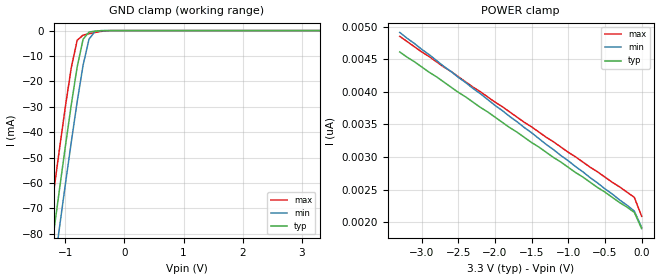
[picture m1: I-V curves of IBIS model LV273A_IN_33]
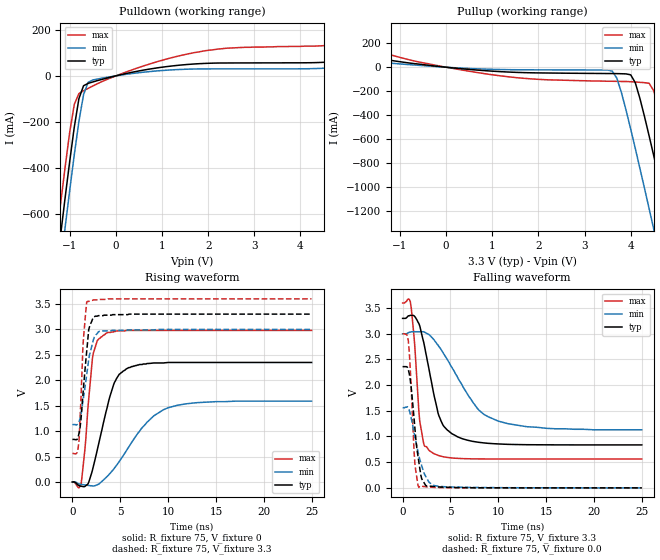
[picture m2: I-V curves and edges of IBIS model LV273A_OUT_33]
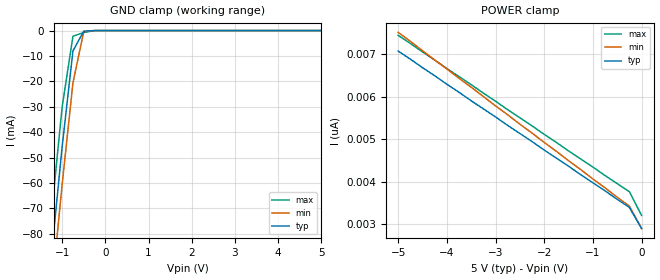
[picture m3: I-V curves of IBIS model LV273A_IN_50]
| TEXAS INSTRUMENTS INCORPORATED
| Standard Linear and Logic Group
| IBIS Model of SN74LV273A
| OCTAL EDGE-TRIGGERED D-TYPE FLIP-FLOP WITH CLEAR
| SOIC 20-pin (DW), SOP 20-pin (NS), SSOP 20-pin (DB), TSSOP 20-pin (PW)
| and TVSOP 20-pin (DGV) Package
[IBIS Ver]   3.2
[Comment Char]  |_char
[File Name]   lv273a.ibs
[File Rev]   2.0 H_die
[Date]   May 29, 2000
[Source]   Data created from HSPICE simulations at TI-SLL.
[Notes]   The following is an IBIS list for the LV273A.
|   Please contact sllibis@ti.com with questions and
|   comments concerning SLL IBIS models.
[Disclaimer] Property of Texas Instruments Incorporated.  Unauthorized
   reproduction and/or distribution is strictly prohibited.
   This product is protected under copyright law.
   Created 2000, (C) Copyright 2000, Texas Instruments Inc.,
   All Rights Reserved.
   UNLESS THERE IS A SIGNED, WRITTEN AGREEMENT TO THE
   CONTRARY, TEXAS INSTRUMENTS () IS PROVIDING THE IBIS
   MODELS  AND WITHOUT ANY WARRANTY, EXPRESSED OR
   IMPLIED.  TI assumes no liability for:
   1) the accuracy of the IBIS models provided to your
   company;
   2) the proper functioning of these IBIS Models in your
   design or for any resulting applications; or
   3) infringement of patents, copyrights or intellectual
   property rights resulting from your use of these IBIS
   models.
   TI provides IBIS Models as a service to our customers.
   You and your company shall not distribute, sell or give
   these models to anyone else without prior written
   permission from TI.
   TI reserves the right to make changes to our products or
   to discontinue any semiconductor product or service
   without notice, and advises our customers to obtain the
   latest version of relevant information to verify, before
   placing orders, that the information being relied on is
   current.
   Please be aware that your receipt and use of the IBIS
   information provided shall serve as acceptance of these
   terms and conditions.  If you do not accept these terms,
   you should return or destroy the IBIS models and any
   other accompanying information immediately.
|   Component LV273A_DW
[Component]   LV273A_DW
[Manufacturer]  Texas Instruments, Inc.
[Package]
|   typ   min   max
R_pkg   0.038   0.033   0.045
L_pkg   5.012nH   4.110nH   6.349nH
C_pkg   0.717pF   0.530pF   0.868pF
[Pin]   signal_name   model_name   R_pin   L_pin   C_pin
1   CLR_NOT   LV273A_IN   0.042   6.336nH   0.865pF
2   1Q   LV273A_OUT   0.043   5.542nH   0.867pF
3   1D   LV273A_IN   0.034   4.714nH   0.732pF
4   2D   LV273A_IN   0.034   4.377nH   0.591pF
5   2Q   LV273A_OUT   0.036   4.130nH   0.533pF
6   3Q   LV273A_OUT   0.035   4.111nH   0.530pF
7   3D   LV273A_IN   0.034   4.284nH   0.583pF
8   4D   LV273A_IN   0.034   4.634nH   0.726pF
9   4Q   LV273A_OUT   0.040   5.518nH   0.865pF
10   GND   GND   0.043   6.349nH   0.866pF
11   CLK   LV273A_IN   0.041   6.281nH   0.861pF
12   5Q   LV273A_OUT   0.045   5.561nH   0.868pF
13   5D   LV273A_IN   0.033   4.778nH   0.742pF
14   6D   LV273A_IN   0.035   4.414nH   0.596pF
15   6Q   LV273A_OUT   0.035   4.110nH   0.533pF
16   7Q   LV273A_OUT   0.036   4.130nH   0.533pF
17   7D   LV273A_IN   0.034   4.377nH   0.591pF
18   8D   LV273A_IN   0.034   4.714nH   0.731pF
19   8Q   LV273A_OUT   0.043   5.569nH   0.868pF
20   VCC   POWER   0.042   6.308nH   0.864pF
|   Component LV273A_NS
[Component]   LV273A_NS
[Manufacturer]  Texas Instruments, Inc.
[Package]
|   typ   min   max
R_pkg   0.044   0.029   0.058
L_pkg   3.666nH   2.317nH   5.115nH
C_pkg   0.548pF   0.316pF   0.725pF
[Pin]   signal_name   model_name   R_pin   L_pin   C_pin
1   CLR_NOT   LV273A_IN   0.058   5.115nH   0.725pF
2   1Q   LV273A_OUT   0.053   4.591nH   0.724pF
3   1D   LV273A_IN   0.049   3.754nH   0.572pF
4   2D   LV273A_IN   0.029   2.549nH   0.388pF
5   2Q   LV273A_OUT   0.031   2.317nH   0.316pF
6   3Q   LV273A_OUT   0.031   2.317nH   0.316pF
7   3D   LV273A_IN   0.029   2.556nH   0.399pF
8   4D   LV273A_IN   0.049   3.754nH   0.579pF
9   4Q   LV273A_OUT   0.053   4.591nH   0.724pF
10   GND   GND   0.058   5.115nH   0.725pF
11   CLK   LV273A_IN   0.058   5.115nH   0.725pF
12   5Q   LV273A_OUT   0.053   4.591nH   0.724pF
13   5D   LV273A_IN   0.049   3.754nH   0.579pF
14   6D   LV273A_IN   0.029   2.557nH   0.399pF
15   6Q   LV273A_OUT   0.031   2.317nH   0.316pF
16   7Q   LV273A_OUT   0.031   2.317nH   0.316pF
17   7D   LV273A_IN   0.029   2.557nH   0.399pF
18   8D   LV273A_IN   0.049   3.754nH   0.579pF
19   8Q   LV273A_OUT   0.053   4.591nH   0.724pF
20   VCC   POWER   0.058   5.115nH   0.725pF
|   Component LV273A_DB
[Component]   LV273A_DB
[Manufacturer]  Texas Instruments, Inc.
[Package]
|   typ   min   max
R_pkg   0.040   0.035   0.051
L_pkg   3.495nH   3.035nH   4.314nH
C_pkg   0.420pF   0.346pF   0.502pF
[Pin]   signal_name   model_name   R_pin   L_pin   C_pin
1   CLR_NOT   LV273A_IN   0.049   4.310nH   0.502pF
2   1Q   LV273A_OUT   0.048   3.903nH   0.487pF
3   1D   LV273A_IN   0.035   3.189nH   0.396pF
4   2D   LV273A_IN   0.035   3.036nH   0.347pF
5   2Q   LV273A_OUT   0.035   3.035nH   0.367pF
6   3Q   LV273A_OUT   0.035   3.035nH   0.367pF
7   3D   LV273A_IN   0.035   3.036nH   0.347pF
8   4D   LV273A_IN   0.035   3.189nH   0.397pF
9   4Q   LV273A_OUT   0.047   3.899nH   0.488pF
10   GND   GND   0.051   4.314nH   0.500pF
11   CLK   LV273A_IN   0.051   4.314nH   0.500pF
12   5Q   LV273A_OUT   0.047   3.899nH   0.488pF
13   5D   LV273A_IN   0.035   3.189nH   0.397pF
14   6D   LV273A_IN   0.035   3.036nH   0.346pF
15   6Q   LV273A_OUT   0.035   3.035nH   0.367pF
16   7Q   LV273A_OUT   0.035   3.035nH   0.367pF
17   7D   LV273A_IN   0.035   3.036nH   0.346pF
18   8D   LV273A_IN   0.035   3.189nH   0.397pF
19   8Q   LV273A_OUT   0.047   3.899nH   0.488pF
20   VCC   POWER   0.051   4.314nH   0.502pF
|   Component LV273A_PW
[Component]   LV273A_PW
[Manufacturer]  Texas Instruments, Inc.
[Package]
|   typ   min   max
R_pkg   0.035   0.024   0.047
L_pkg   2.399nH   1.710nH   3.250nH
C_pkg   0.284pF   0.166pF   0.418pF
[Pin]   signal_name   model_name   R_pin   L_pin   C_pin
1   CLR_NOT   LV273A_IN   0.041   3.102nH   0.410pF
2   1Q   LV273A_OUT   0.040   2.777nH   0.363pF
3   1D   LV273A_IN   0.029   2.194nH   0.260pF
4   2D   LV273A_IN   0.025   1.710nH   0.166pF
5   2Q   LV273A_OUT   0.025   1.740nH   0.191pF
6   3Q   LV273A_OUT   0.024   1.763nH   0.193pF
7   3D   LV273A_IN   0.024   1.817nH   0.174pF
8   4D   LV273A_IN   0.028   2.256nH   0.265pF
9   4Q   LV273A_OUT   0.045   2.887nH   0.368pF
10   GND   GND   0.047   3.250nH   0.417pF
11   CLK   LV273A_IN   0.046   3.244nH   0.418pF
12   5Q   LV273A_OUT   0.046   2.961nH   0.375pF
13   5D   LV273A_IN   0.033   2.334nH   0.268pF
14   6D   LV273A_IN   0.029   1.915nH   0.179pF
15   6Q   LV273A_OUT   0.031   1.934nH   0.203pF
16   7Q   LV273A_OUT   0.032   1.917nH   0.201pF
17   7D   LV273A_IN   0.030   1.833nH   0.173pF
18   8D   LV273A_IN   0.036   2.324nH   0.268pF
19   8Q   LV273A_OUT   0.042   2.869nH   0.372pF
20   VCC   POWER   0.042   3.160nH   0.414pF
|   Component LV273A_DGV
[Component]   LV273A_DGV
[Manufacturer]  Texas Instruments, Inc.
[Package]
|   typ   min   max
R_pkg   0.044   0.038   0.048
L_pkg   2.561nH   2.236nH   2.961nH
C_pkg   0.342pF   0.264pF   0.446pF
[Pin]   signal_name   model_name   R_pin   L_pin   C_pin
1   CLR_NOT   LV273A_IN   0.044   2.935nH   0.417pF
2   1Q   LV273A_OUT   0.042   2.869nH   0.446pF
3   1D   LV273A_IN   0.043   2.399nH   0.316pF
4   2D   LV273A_IN   0.044   2.236nH   0.265pF
5   2Q   LV273A_OUT   0.046   2.278nH   0.264pF
6   3Q   LV273A_OUT   0.045   2.274nH   0.264pF
7   3D   LV273A_IN   0.044   2.285nH   0.269pF
8   4D   LV273A_IN   0.043   2.452nH   0.320pF
9   4Q   LV273A_OUT   0.044   2.900nH   0.446pF
10   GND   GND   0.044   2.961nH   0.418pF
11   CLK   LV273A_IN   0.045   2.954nH   0.418pF
12   5Q   LV273A_OUT   0.042   2.847nH   0.443pF
13   5D   LV273A_IN   0.045   2.453nH   0.319pF
14   6D   LV273A_IN   0.045   2.297nH   0.269pF
15   6Q   LV273A_OUT   0.048   2.334nH   0.268pF
16   7Q   LV273A_OUT   0.048   2.335nH   0.267pF
17   7D   LV273A_IN   0.046   2.299nH   0.268pF
18   8D   LV273A_IN   0.046   2.457nH   0.320pF
19   8Q   LV273A_OUT   0.043   2.848nH   0.441pF
20   VCC   POWER   0.038   2.812nH   0.408pF
[Model Selector]   LV273A_IN
LV273A_IN_33   3.3-V Vcc Input Model
LV273A_IN_50   5.0-V Vcc Input Model
[Model Selector]   LV273A_OUT
LV273A_OUT_33   3.3-V Vcc Output Model
LV273A_OUT_50   5.0-V Vcc Output Model
| Models and submodels in the file (4): LV273A_IN_33 (Input), LV273A_OUT_33 (Output), LV273A_IN_50 (Input), LV273A_OUT_50 (Output)
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|   Model LV273A_IN_33
[Model]   LV273A_IN_33
Model_type  Input
Polarity   Inverting
Vinl = 0.99
Vinh = 2.31
| variable   typ   min   max
C_comp   1.43pf   1.07pf   1.79pf
[Temperature Range]   25   85   -40
[Voltage Range]   3.3   3.0   3.6
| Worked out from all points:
|   GND clamp passes 1 mA (typ) near -0.61 V on its own axis
[GND Clamp]
|   Voltage   I(typ)   I(min)   I(max)
-3.3V     -460mA     -475mA     -445mA
-1.3V     -97.5mA    -113mA     -81.5mA
-1.2V     -79.9mA    -95mA      -63.9mA
-1.1V     -62.6mA    -77.6mA    -46.7mA
-1V       -45.6mA    -60.5mA    -30mA
-900mV    -29.2mA    -43.9mA    -14.6mA
-800mV    -14.3mA    -28mA      -3.81mA
-700mV    -3.42mA    -13.6mA    -1.78mA
-600mV    -581uA     -3.4mA     -1.25mA
-500mV    -233uA     -353uA     -759uA
-400mV    -58.1uA    -21.9uA    -324uA
3.3V      1.9nA      2.34nA     1.69nA
[POWER Clamp]
|   Voltage   I(typ)   I(min)   I(max)
-3.3V     4.61nA     4.91nA     4.85nA
-3V       4.38nA     4.65nA     4.61nA
-100mV    2.15nA     2.17nA     2.38nA
0V        1.9nA      1.92nA     2.09nA
|   Model LV273A_OUT_33
[Model]   LV273A_OUT_33
Model_type  Output
Polarity   Non-Inverting
Vmeas = 1.65v
Cref = 15pf
| variable   typ   min   max
C_comp   7.60pf   5.70pf   9.50pf
[Temperature Range]   25   85   -40
[Voltage Range]   3.3   3.0   3.6
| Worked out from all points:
|   slope of the pulldown table from 0 to 0.495 V, typ, clamps not added: 23.3 ohm
|   slope of the pullup table from 0 to 0.495 V, typ, clamps not added: 27.2 ohm
|   rising waveform, R_fixture 75, V_fixture 0: 20-80 % time 1.85ns typ, 3.78ns min, 791ps max; typ from 0 V to 2.35 V
|   falling waveform, R_fixture 75, V_fixture 3.3: 20-80 % time 1.73ns typ, 3.79ns min, 738ps max; typ from 3.3 V to 0.836 V
|   rising waveform, R_fixture 75, V_fixture 3.3: 20-80 % time 676ps typ, 932ps min, 452ps max; typ from 0.836 V to 3.3 V
|   falling waveform, R_fixture 75, V_fixture 0.0: 20-80 % time 791ps typ, 1.17ns min, 463ps max; typ from 2.36 V to 0 V
[Pulldown]
|   Voltage   I(typ)   I(min)   I(max)
-3.3V     -4.35A     -4.47A     -4.22A
-1.3V     -864mA     -992mA     -728mA
-1.2V     -696mA     -825mA     -560mA
-1.1V     -531mA     -660mA     -398mA
-900mV    -222mA     -342mA     -124mA
-800mV    -99mA      -198mA     -76.7mA
-700mV    -42.9mA    -81.7mA    -64.5mA
-600mV    -32.5mA    -27.9mA    -54.3mA
-500mV    -26.5mA    -17.9mA    -44.1mA
1.9V      53.8mA     30.3mA     108mA
4.9V      64.5mA     37.1mA     138mA
6.6V      104mA      62.3mA     203mA
[Pullup]
|   Voltage   I(typ)   I(min)   I(max)
-3.3V     168mA      93.3mA     315mA
600mV     -21.6mA    -12.3mA    -39.7mA
3.6V      -52.9mA    -32mA      -117mA
3.7V      -53.4mA    -91mA      -118mA
4V        -63.3mA    -515mA     -121mA
4.2V      -260mA     -843mA     -126mA
4.4V      -573mA     -1.18A     -134mA
4.5V      -738mA     -1.35A     -197mA
4.8V      -1.25A     -1.87A     -656mA
4.9V      -1.42A     -2.04A     -825mA
5.2V      -1.94A     -2.56A     -1.34A
6.6V      -4.39A     -5.02A     -3.79A
[Ramp]
| variable   typ   min   max
dV/dt_r   1.42E+00/1.85E-09   9.64E-01/3.85E-09   1.79E+00/7.65E-10
dV/dt_f   1.52E+00/1.74E-09   1.15E+00/3.88E-09   1.87E+00/7.16E-10
R_load = 75
[Rising Waveform]
R_fixture = 75
V_fixture = 0
|   Time   V(typ)   V(min)   V(max)
0s        0V         0V         0V
900ps     -82mV      -46.7mV    -50.3mV
1.3ns     -86.7mV    -56.2mV    630mV
2.1ns     238mV      -76.1mV    2.44V
2.6ns     632mV      -53.1mV    2.78V
3.5ns     1.37V      86.1mV     2.92V
4.9ns     2.12V      405mV      2.97V
7.8ns     2.33V      1.18V      2.98V
10ns      2.35V      1.46V      2.98V
25ns      2.35V      1.59V      2.98V
[Falling Waveform]
R_fixture = 75
V_fixture = 3.3
V_fixture_min = 3.0
V_fixture_max = 3.6
|   Time   V(typ)   V(min)   V(max)
0s        3.3V       3V         3.6V
800ps     3.36V      3.03V      3.63V
1.2ns     3.35V      3.04V      2.94V
1.8ns     3.15V      3.04V      1.29V
2.3ns     2.75V      3.03V      810mV
3.2ns     1.88V      2.9V       674mV
3.8ns     1.4V       2.75V      627mV
4.7ns     1.12V      2.49V      592mV
9ns       866mV      1.38V      562mV
25ns      836mV      1.13V      562mV
[Rising Waveform]
R_fixture = 75
V_fixture = 3.3
V_fixture_min = 3.0
V_fixture_max = 3.6
|   Time   V(typ)   V(min)   V(max)
0s        836mV      1.13V      562mV
500ps     839mV      1.13V      581mV
700ps     965mV      1.19V      831mV
900ps     1.24V      1.34V      1.66V
1.1ns     1.72V      1.59V      2.68V
1.5ns     2.58V      2.12V      3.54V
1.8ns     3.06V      2.51V      3.56V
2.3ns     3.25V      2.85V      3.58V
2.8ns     3.27V      2.96V      3.59V
25ns      3.3V       3V         3.6V
[Falling Waveform]
R_fixture = 75
V_fixture = 0.0
|   Time   V(typ)   V(min)   V(max)
0s        2.36V      1.56V      3V
600ps     2.3V       1.56V      2.86V
800ps     2.1V       1.44V      2.32V
1.2ns     1.35V      1.07V      703mV
1.3ns     1.13V      979mV      433mV
1.7ns     502mV      626mV      8.38mV
2ns       175mV      430mV      32.2mV
2.4ns     51mV       228mV      21.5mV
3.7ns     18.8mV     32.1mV     6.62mV
25ns      0V         26.4uV     5.59uV
|   Model LV273A_IN_50
[Model]   LV273A_IN_50
Model_type  Input
Polarity   Inverting
Vinl = 1.5
Vinh = 3.5
| variable   typ   min   max
C_comp   1.43pf   1.07pf   1.79pf
[Temperature Range]   25   85   -40
[Voltage Range]   5.0   4.5   5.5
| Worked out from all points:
|   GND clamp passes 1 mA (typ) near -0.52 V on its own axis
[GND Clamp]
|   Voltage   I(typ)   I(min)   I(max)
-5V       -773mA     -786mA     -758mA
-1.5V     -133mA     -148mA     -117mA
-1.25V    -88.7mA    -104mA     -72.7mA
-1V       -45.6mA    -60.5mA    -30mA
-750mV    -7.99mA    -20.5mA    -2.23mA
-500mV    -233uA     -353uA     -759uA
-250mV    -2.63nA    -182nA     -26.9uA
5V        2.9nA      3.64nA     2.54nA
[POWER Clamp]
|   Voltage   I(typ)   I(min)   I(max)
-5V       7.08nA     7.52nA     7.45nA
-1.5V     4.37nA     4.5nA      4.73nA
-250mV    3.4nA      3.43nA     3.77nA
0V        2.9nA      2.91nA     3.21nA
